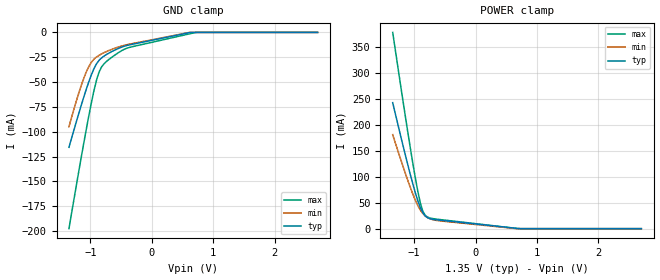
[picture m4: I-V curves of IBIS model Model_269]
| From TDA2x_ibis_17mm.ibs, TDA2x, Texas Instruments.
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| Model based on original model for DDR_SEIOPB_H
|   Sub model DDR3L_ODT_80_1P35
[model]   Model_269
|[Description]  [1.35V-INPUT-X-X]
|   , ,
|[Input Load]
|[Output Drive]
|Voltage   1.35V
|Mode   INPUT
Model_type   Input
Polarity   Non-Inverting
Vinl = 0.585
Vinh = 0.765
C_comp   1p   0.5p   1.75p
[Receiver Thresholds]
Tslew_ac = 5n
Vth= 0.675
Vth_max= 0.709
Vth_min= 0.608
Vinh_ac= 0.175
Vinh_dc= 0.1
Vinl_ac= -0.175
Vinl_dc= -0.1
[Temperature Range]   25   125   -40
[Voltage Range]   1.35   1.2825   1.4175
[POWER_clamp]
-1.35V    242.9mA    181.2mA    378.4mA
-1.145V   142.6mA    107mA      217.7mA
-1.064V   104.6mA    79.6mA     156mA
-981.8mV  69.39mA    54.98mA    98.09mA
-940.9mV  53.78mA    44.47mA    71.92mA
-900mV    40.49mA    35.74mA    49.52mA
-859.1mV  30.56mA    29.07mA    33.54mA
-818.2mV  24.29mA    24.28mA    25.28mA
-736.4mV  19.06mA    18.69mA    20.43mA
-613.6mV  16.66mA    15.53mA    18.01mA
695.5mV   302.9uA    0A         33.14uA
2.7V      0A         0A         0A
[GND_clamp]
-1.35V    -115.6mA   -94.89mA   -197.5mA
-1.227V   -89.36mA   -68.54mA   -153.1mA
-1.105V   -64.31mA   -45.5mA    -110mA
-1.023V   -49.02mA   -33.92mA   -82.75mA
-940.9mV  -36.24mA   -26.85mA   -58.09mA
-859.1mV  -28.07mA   -23.04mA   -39.84mA
-777.3mV  -23.77mA   -20.37mA   -31.48mA
-695.5mV  -20.72mA   -18.12mA   -27.05mA
-368.2mV  -12.61mA   -11.9mA    -15.17mA
613.6mV   -211.8uA   -17.74uA   -1.47mA
736.4mV   0A         0A         0A
2.7V      0A         0A         0A
